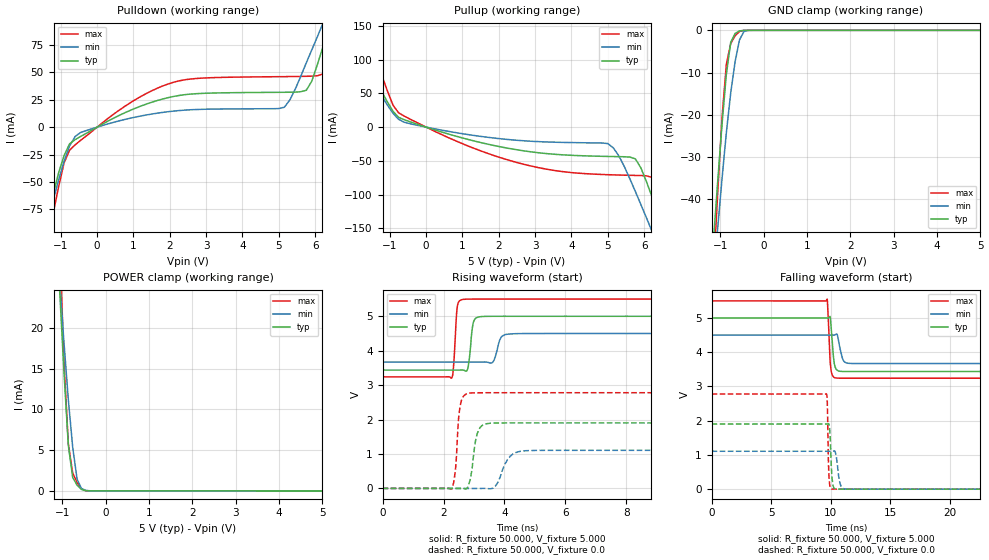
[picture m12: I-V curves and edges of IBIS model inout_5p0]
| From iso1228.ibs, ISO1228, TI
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|   Model inout_5p0
[Model] inout_5p0
Model_type I/O
Vinl =  1.500V
Vinh =  3.500V
Polarity   Non-Inverting
Enable   Active-High
Vmeas = 2.5
Vref = 0
Cref = 15pF
Rref = 1000
C_comp   0.978pF   1.050pF   0.889pF
[Model Spec]
Vinh   3.500V   3.150V   3.850V
Vinl   1.500V   1.350V   1.650V
[Temperature Range]   27.000   0.150k   -40.000
[Voltage Range]   5.000V   4.500V   5.500V
[Pullup Reference]   5.000V   4.500V   5.500V
[Pulldown Reference]   0.0V   0.0V   0.0V
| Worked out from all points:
|   slope of the pulldown table from 0 to 0.75 V, typ, clamps not added: 58.1 ohm
|   slope of the pullup table from 0 to 0.75 V, typ, clamps not added: 60.7 ohm
|   GND clamp passes 1 mA (typ) near -0.67 V on its own axis
|   POWER clamp passes 1 mA (typ) near -0.69 V on its own axis
|   rising waveform, R_fixture 50.000, V_fixture 5.000: 20-80 % time 106ps typ, 155ps min, 85.7ps max; typ from 3.44 V to 5 V
|   rising waveform, R_fixture 50.000, V_fixture 0.0: 20-80 % time 187ps typ, 333ps min, 126ps max; typ from 0 V to 1.9 V
|   falling waveform, R_fixture 50.000, V_fixture 5.000: 20-80 % time 227ps typ, 317ps min, 176ps max; typ from 5 V to 3.44 V
|   falling waveform, R_fixture 50.000, V_fixture 0.0: 20-80 % time 143ps typ, 253ps min, 98.5ps max; typ from 1.9 V to 0 V
[Pulldown]
|Voltage   I(typ)   I(min)   I(max)
-5V       -815.5mA   -672.8mA   -1.202A
-1.515V   -105.6mA   -105.1mA   -136.1mA
-1.212V   -61.35mA   -66.74mA   -79.03mA
-909mV    -25.88mA   -31.11mA   -32.53mA
-606mV    -11.4mA    -8.566mA   -16.16mA
1.212V    19.31mA    10.22mA    28.12mA
5.152V    31.78mA    18.16mA    46.05mA
5.758V    33.62mA    58.73mA    46.36mA
6.212V    72.89mA    94.39mA    48.42mA
6.364V    89.22mA    106.5mA    53.15mA
6.667V    121.6mA    131.9mA    95.16mA
10V       660.1mA    546.8mA    912.1mA
[Pullup]
|Voltage   I(typ)   I(min)   I(max)
-5V       644mA      477.1mA    1.049A
-2.424V   204.2mA    153.2mA    323.8mA
-2.121V   160.1mA    122.2mA    245mA
-1.667V   102.5mA    83.45mA    148.2mA
-758mV    14.58mA    11.61mA    21.29mA
2.273V    -31.52mA   -18.45mA   -49.05mA
5V        -43.5mA    -24.42mA   -70.59mA
5.758V    -47.03mA   -95.47mA   -71.69mA
6.212V    -102.6mA   -154mA     -74.33mA
6.515V    -148.3mA   -193.8mA   -102.8mA
6.818V    -195mA     -237.4mA   -163.6mA
10V       -864.2mA   -796.2mA   -1.115A
[GND_clamp]
|Voltage   I(typ)   I(min)   I(max)
-5V       -814.6mA   -672.4mA   -1.2A
-1.162V   -50.63mA   -59.51mA   -58.77mA
-1.061V   -36.17mA   -47.19mA   -38.95mA
-960mV    -22.43mA   -35.32mA   -20.84mA
-859mV    -10.4mA    -24.25mA   -8.047mA
-758mV    -2.819mA   -14.8mA    -3.107mA
-657mV    -734.5uA   -7.403mA   -1.295mA
-556mV    -143.3uA   -2.276mA   -265.4uA
-455mV    -10.51uA   -285uA     -11.72uA
-354mV    -1.087uA   -24.14uA   -1.065uA
5V        0A         0A         0A
[POWER_clamp]
|Voltage   I(typ)   I(min)   I(max)
-5V       612mA      452.6mA    1.004A
-1.061V   24.81mA    26mA       31.08mA
-960mV    14.69mA    18.27mA    15.96mA
-859mV    5.613mA    11.21mA    5.802mA
-758mV    1.648mA    5.353mA    2.188mA
-657mV    709.3uA    1.442mA    1.033mA
-556mV    189.6uA    309.5uA    237.7uA
-455mV    24.33uA    61.5uA     22.71uA
-354mV    11.34uA    14.21uA    15.25uA
5V        0A         0A         1.293uA
[Ramp]
| variable   typ   min   max
dV/dt_r   1.142/0.185n   0.664/0.334n   1.668/0.127n
dV/dt_f   0.938/0.224n   0.498/0.314n   1.355/0.180n
R_load = 50.000
[Rising Waveform]
R_fixture= 50.000
V_fixture= 5.000
V_fixture_min= 4.500
V_fixture_max= 5.500
|time   V(typ)   V(min)   V(max)
0s        3.437V     3.67V      3.241V
2.27ns    3.437V     3.67V      3.207V
2.46ns    3.437V     3.67V      5.317V
2.79ns    3.464V     3.67V      5.498V
3ns       4.873V     3.67V      5.5V
3.4ns     4.998V     3.67V      5.5V
3.62ns    4.999V     3.669V     5.5V
3.92ns    5V         4.418V     5.5V
4.64ns    5V         4.498V     5.5V
100ns     5V         4.5V       5.5V
[Rising Waveform]
R_fixture= 50.000
V_fixture= 0.0
V_fixture_min= 0.0
V_fixture_max= 0.0
|time   V(typ)   V(min)   V(max)
0s        3.3nV      128.9nV    17.73nV
2.26ns    181.6nV    128.7nV    -19.16mV
2.39ns    -18.36uV   121.2nV    532.5mV
2.55ns    399.7uV    -199.8nV   2.418V
2.81ns    69.52mV    1.806uV    2.76V
2.98ns    925.7mV    -17.58uV   2.776V
3.31ns    1.852V     728.1uV    2.779V
4.27ns    1.902V     996.7mV    2.779V
5.07ns    1.902V     1.105V     2.779V
100ns     1.903V     1.107V     2.779V
[Falling Waveform]
R_fixture= 50.000
V_fixture= 5.000
V_fixture_min= 4.500
V_fixture_max= 5.500
|time   V(typ)   V(min)   V(max)
0s        5V         4.5V       5.5V
9.7ns     4.999V     4.5V       5.553V
9.77ns    4.998V     4.5V       5.209V
9.95ns    5.042V     4.5V       3.786V
10.03ns   4.772V     4.5V       3.488V
10.31ns   3.656V     4.501V     3.263V
10.56ns   3.471V     4.508V     3.244V
11.06ns   3.439V     3.764V     3.241V
11.81ns   3.437V     3.671V     3.241V
100ns     3.437V     3.67V      3.241V
[Falling Waveform]
R_fixture= 50.000
V_fixture= 0.0
V_fixture_min= 0.0
V_fixture_max= 0.0
|time   V(typ)   V(min)   V(max)
0s        1.903V     1.107V     2.779V
9.63ns    1.902V     1.107V     2.787V
9.72ns    1.902V     1.107V     2.524V
9.81ns    1.91V      1.107V     869.6mV
9.86ns    1.896V     1.107V     368.3mV
10.18ns   147.1mV    1.108V     2.905mV
10.43ns   7.146mV    1.032V     681.5uV
10.82ns   513.6uV    131mV      190.8uV
11.29ns   154.1uV    3.587mV    47.38uV
100ns     62.93nV    170.1nV    61.69nV
